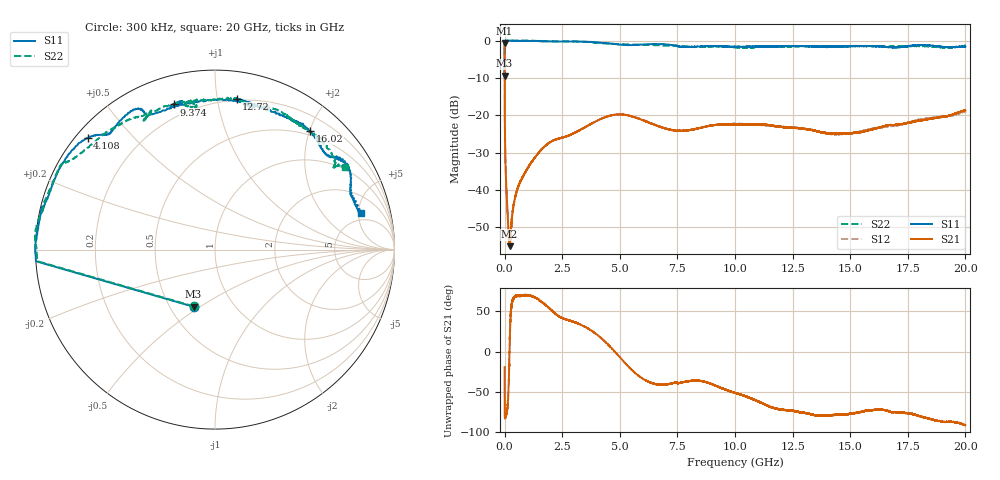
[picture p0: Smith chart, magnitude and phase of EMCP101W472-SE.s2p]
!EMCP101W472
!Johanson Technology Inc.
!www.johansontechnology.com
!Test Board Conditions:
!Substrate Type  RO4350B
!Substrate Thickness  10 mil
!Substrate Dk  3.66
!TL Type: GCPW
!TL Trace Width  20 mil
!TL Gap  10 mil
!PART MODE SINGLE ENDED (AKA BYPASS)
!DUT TOPOLOGY	SERIES-SHUNT
# MHz S  dB  R 50
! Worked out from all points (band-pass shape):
!   20001 points, 300 kHz to 20 GHz, reference 50 ohm
!   highest |S21| = -0.59 dB at 300 kHz (marker M1); lowest = -55.0 dB at 213.3 MHz (marker M2)
!   |S21| within 3 dB of the highest: start of sweep to 933.2 kHz
!   lowest |S11| = -9.4 dB at 300 kHz (marker M3), VSWR 2.03, Z = 32.7 - j23.5 ohm
!   |S11| at or under -10 dB: nowhere
!   |S22| runs from -9.4 to 0.1 dB; largest |S21 - S12| = 0.0066
!   S11 on the Smith chart (normalised r, x): 300 kHz: 0.65, -0.47; 4.108 GHz: 0.03, +0.38; 9.374 GHz: 0.14, +0.75; 12.72 GHz: 0.19, +1.14; 16.02 GHz: 0.43, +2.01; 20 GHz: 3.89, +5.29
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0.3  -9.37 -110.5  -0.59 -19.5  -0.57 -19.5  -9.43 -110.7
112.298  0.02 179.4  -44.05 -72.4  -44.13 -72.8  -0.04 179.9
159.298  0.01 178.9  -50.10 -54.7  -50.04 -56.7  -0.02 179.6
213.297  0.01 178.4  -55.02 -1.3  -54.67 -2.3  -0.03 179.1
566.292  -0.04 174.8  -39.61 69.7  -39.52 69.3  0.03 176.9
1198.282  -0.08 168.7  -32.24 69.0  -32.29 69.2  -0.00 170.9
1956.271  -0.17 164.5  -27.27 53.5  -27.18 53.5  -0.18 158.8
3334.25  -0.24 147.6  -23.70 33.0  -23.72 33.1  -0.25 150.2
4108.238  -0.50 138.7  -21.16 18.9  -21.13 18.8  -0.61 146.7
5175.222  -1.12 133.2  -19.82 -12.6  -19.84 -12.4  -0.97 135.5
6667.2  -0.89 120.3  -22.88 -41.1  -22.82 -41.4  -1.22 123.6
7600.186  -1.59 115.1  -24.12 -39.0  -24.12 -39.0  -1.43 115.0
8509.172  -1.50 103.3  -23.35 -36.6  -23.31 -37.0  -1.66 118.2
9374.159  -1.51 105.9  -22.43 -45.0  -22.46 -44.2  -1.44 104.8
10000.15  -1.62 106.1  -22.43 -51.3  -22.25 -51.2  -1.76 97.6
11358.13  -1.56 82.0  -22.53 -66.8  -22.70 -66.9  -1.53 100.1
12715.11  -1.44 81.9  -23.39 -74.5  -23.31 -74.9  -1.45 86.8
13334.1  -1.55 76.0  -23.89 -78.3  -23.87 -78.7  -1.50 80.0
14418.08  -1.54 60.3  -24.95 -78.5  -25.06 -78.7  -1.62 73.8
16021.06  -1.46 51.3  -23.67 -72.7  -23.58 -74.3  -1.49 59.7
16667.05  -1.75 43.3  -22.57 -74.4  -22.86 -74.7  -1.53 57.2
20000  -1.55 14.1  -18.61 -91.9  -18.94 -90.3  -1.29 32.3
